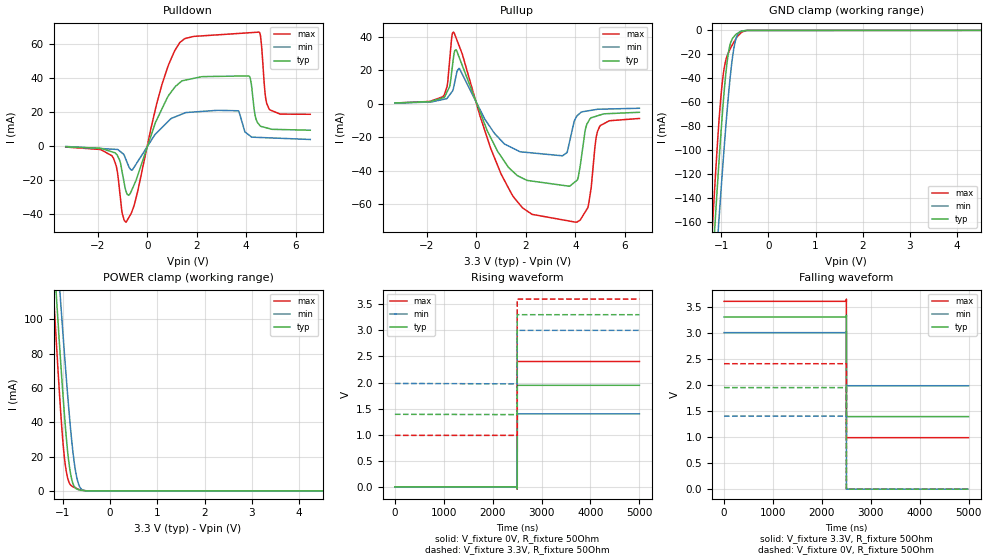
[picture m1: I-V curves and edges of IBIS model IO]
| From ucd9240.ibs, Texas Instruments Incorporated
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|   IO 3.3V Model
[Model]   IO
Model_type   I/O
|Signals
Vinl =  0.65V
Vinh =  2.85V
Vmeas = 1.475V
Vref = 3.3V
|Rref = 50Ohm
| variable   typ   min   max
|C_comp Output Disabled   (NOM PVT)   (FAST PVT)   (SLOW PVT)
C_comp   1.475pF   1.443pF   1.508pF
|C_comp Output Low   (NOM PVT)   (SLOW PVT)   (FAST PVT)
|C_comp   2.352pF   2.12pF   2.485pF
|C_comp Output High   (NOM PVT)   (SLOW PVT)   (FAST PVT)
|C_comp   3.588pF   4.366pF   11.333pF
|Junction Temperature
[Temperature Range]   27.0   110.0   -40.0
[Voltage range]   3.3V   3.0V   3.6V
[pullup reference]   3.3V   3.0V   3.6V
[power clamp reference]   3.3V   3.0V   3.6V
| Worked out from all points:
|   slope of the pulldown table from 0 to 0.495 V, typ, clamps not added: 25.7 ohm
|   slope of the pullup table from 0 to 0.495 V, typ, clamps not added: 26.7 ohm
|   GND clamp passes 1 mA (typ) near -0.59 V on its own axis
|   POWER clamp passes 1 mA (typ) near -0.70 V on its own axis
|   falling waveform, V_fixture 3.3V, R_fixture 50Ohm: 20-80 % time 340ps typ, 421ps min, 207ps max; typ from 3.3 V to 1.39 V
|   rising waveform, V_fixture 0V, R_fixture 50Ohm: 20-80 % time 708ps typ, 1.32ns min, 449ps max; typ from 0 V to 1.95 V
|   rising waveform, V_fixture 3.3V, R_fixture 50Ohm: 20-80 % time 191ps typ, 179ps min, 136ps max; typ from 1.39 V to 3.3 V
|   falling waveform, V_fixture 0V, R_fixture 50Ohm: 20-80 % time 137ps typ, 200ps min, 87.7ps max; typ from 1.95 V to 0 V
[Pulldown]
|   Voltage   I(typ)   I(min)   I(max)
-3.3V     -501.7uA   -306.3uA   -648.9uA
-1.433V   -3.458mA   -1.887mA   -5.754mA
-867.3mV  -26.36mA   -7.887mA   -44.81mA
-598.8mV  -24.93mA   -13.94mA   -37.54mA
822.5mV   28.76mA    14.15mA    46.26mA
1.862V    39.67mA    19.93mA    64.32mA
3.681V    41.06mA    20.66mA    66.09mA
4.103V    41.15mA    6.486mA    66.49mA
4.526V    12.46mA    4.989mA    66.9mA
4.785V    10.76mA    4.84mA     28.27mA
4.923V    10.23mA    4.76mA     21.76mA
6.59V     9.23mA     3.797mA    18.61mA
[GND Clamp]
|   Voltage   I(typ)   I(min)   I(max)
-3.3V     -1.646A    -1.552A    -1.764A
-1.199V   -203.9mA   -245.2mA   -173.1mA
-1.164V   -181.5mA   -224.8mA   -148.7mA
-1.141V   -167.2mA   -211.4mA   -133.2mA
-1.119V   -153.7mA   -198.7mA   -119mA
-1.055V   -114.3mA   -162mA     -79.87mA
-952.2mV  -57.94mA   -105.5mA   -35.44mA
-847.3mV  -18.71mA   -54.52mA   -18.74mA
-733.4mV  -5.448mA   -15.18mA   -9.859mA
-669.8mV  -2.845mA   -4.95mA    -5.896mA
-590.3mV  -995.3uA   -1.043mA   -2.432mA
6.59V     0A         0A         0A
[Pullup]
|   Voltage   I(typ)   I(min)   I(max)
-3.3V     518.1uA    447.8uA    523.7uA
-1.363V   3.577mA    2.608mA    4.23mA
-1.19V    7.157mA    3.3mA      10.35mA
-932.3mV  27.47mA    9.295mA    42.97mA
-688.4mV  27.43mA    21.03mA    34.24mA
551.3mV   -19.46mA   -13.8mA    -25.62mA
1.43V     -39.88mA   -26.22mA   -54.12mA
3.485V    -48.74mA   -31.03mA   -69.42mA
4.008V    -46.42mA   -8.697mA   -70.8mA
4.508V    -11.06mA   -4.178mA   -62.05mA
4.98V     -6.738mA   -3.186mA   -13.6mA
6.59V     -5.03mA    -2.61mA    -8.729mA
[POWER Clamp]
|   Voltage   I(typ)   I(min)   I(max)
-3.3V     1.126A     1.059A     1.206A
-1.199V   139.3mA    169mA      114.3mA
-1.141V   114.2mA    146mA      86.88mA
-1.055V   77.88mA    112.5mA    48.83mA
-987.2mV  51.21mA    86.79mA    24.19mA
-947.1mV  36.9mA     72.18mA    14.51mA
-835.6mV  9.528mA    35.24mA    3.429mA
-759mV    2.557mA    16.12mA    2.066mA
-698.2mV  955.7uA    6.78mA     1.273mA
-621.5mV  370.3uA    1.374mA    619.3uA
-479.9mV  32.37uA    36uA       50.4uA
6.59V     0A         0A         0A
[Ramp]
R_load = 50
|   typ   min   max
dV/dt_r   1.16808/7.01565e-010  0.840176/1.30988e-009   1.44243/4.42526e-010
dV/dt_f   1.14541/3.06636e-010  0.610549/4.09332e-010   1.56775/2.07614e-010
[Falling Waveform]
V_fixture = 3.3V
V_fixture_min = 3V
V_fixture_max = 3.6V
R_fixture = 50Ohm
C_fixture = 0F
|   Time   V(typ)   V(min)   V(max)
0s        3.3V       3V         3.6V
2.502us   3.308V     3.009V     3.644V
2.502us   3.316V     3.011V     3.439V
2.503us   3.321V     3.015V     2.204V
2.503us   2.898V     3.018V     1.506V
2.503us   2.466V     3.021V     1.156V
2.503us   1.956V     3.025V     1.042V
2.503us   1.565V     2.846V     1V
2.504us   1.399V     2.081V     987.3mV
5us       1.391V     1.982V     987.1mV
[Rising Waveform]
V_fixture = 0V
V_fixture_min = 0V
V_fixture_max = 0V
R_fixture = 50Ohm
C_fixture = 0F
|   Time   V(typ)   V(min)   V(max)
0s        1.029nV    2.401nV    778.6pV
2.502us   -10.87mV   408uV      -44.42mV
2.502us   -26.14mV   408uV      104.1mV
2.502us   43.66mV    -10.02mV   738.4mV
2.502us   582.6mV    3.087mV    1.795V
2.503us   1.015V     122mV      2.197V
2.503us   1.768V     625.1mV    2.383V
2.504us   1.934V     1.233V     2.404V
2.509us   1.947V     1.4V       2.404V
5us       1.947V     1.4V       2.404V
[Rising Waveform]
V_fixture = 3.3V
V_fixture_min = 3V
V_fixture_max = 3.6V
R_fixture = 50Ohm
C_fixture = 0F
|   Time   V(typ)   V(min)   V(max)
0s        1.391V     1.982V     987.1mV
2.501us   1.385V     1.974V     984.7mV
2.502us   1.385V     1.974V     1.214V
2.502us   1.554V     1.974V     2.479V
2.502us   1.72V      1.974V     2.965V
2.502us   2.745V     1.989V     3.501V
2.502us   3.171V     2.195V     3.567V
2.502us   3.29V      2.926V     3.581V
2.503us   3.299V     2.997V     3.6V
5us       3.3V       3V         3.6V
[Falling Waveform]
|Gnd
V_fixture = 0V
V_fixture_min = 0V
V_fixture_max = 0V
R_fixture = 50Ohm
C_fixture = 0F
|   Time   V(typ)   V(min)   V(max)
0s        1.947V     1.4V       2.404V
2.502us   1.948V     1.403V     2.408V
2.502us   1.95V      1.404V     2.35V
2.502us   1.939V     1.405V     1.995V
2.503us   1.759V     1.407V     382.1mV
2.503us   1.538V     1.407V     76.77mV
2.503us   310.2mV    1.4V       8.565mV
2.503us   70.21mV    1.374V     7.504mV
2.503us   31.71mV    70.54mV    146.2uV
5us       1.594nV    3.379nV    1.137nV
